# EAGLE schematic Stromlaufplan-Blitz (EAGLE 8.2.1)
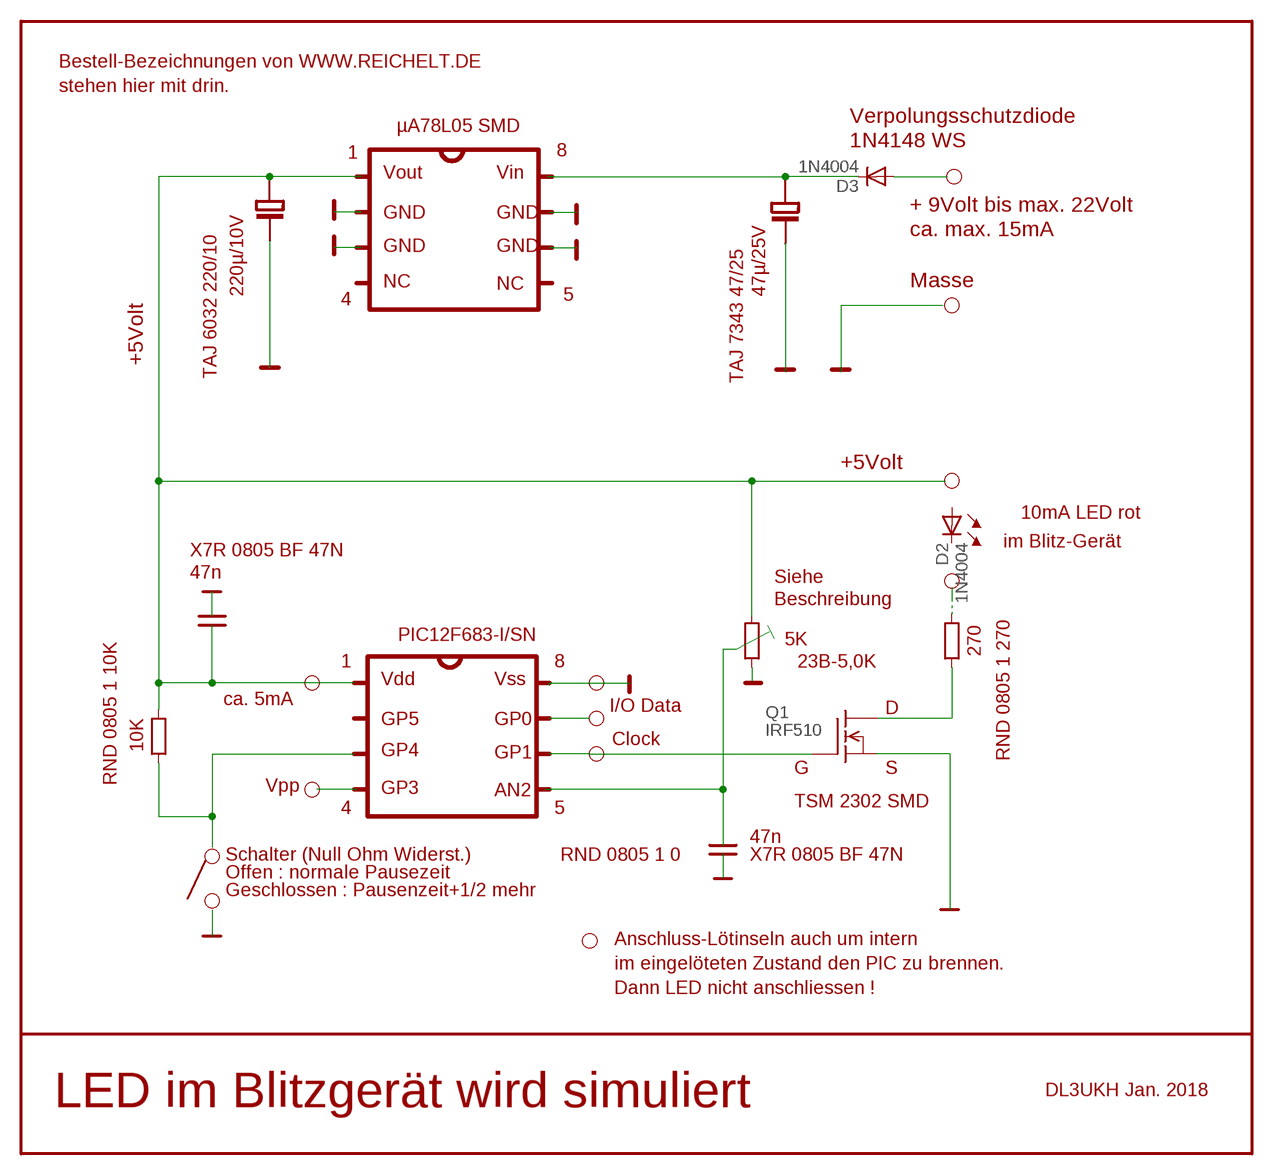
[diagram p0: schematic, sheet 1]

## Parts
D2  1N4004  [DO41-10]
D3  1N4004  [DO41-10]
Q1  IRF510  [TO220]

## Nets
N$5: Q1.1(G)
N$8: Q1.2(D)
N$11: D3.A
N$13: Q1.3(S)
N$35: D3.C
Unconnected: D2.A D2.C

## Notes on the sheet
- Bestell-Bezeichnungen von WWW.REICHELT.DE
- stehen hier mit drin.
- Verpolungsschutzdiode
- µA78L05 SMD
- 1N4148 WS
- 1 | 8
- Vout | Vin
- + 9Volt bis max. 22Volt
- GND | GND
- ca. max. 15mA
- GND | GND
- NC | NC | Masse
- 220µ/10V | 5 | 47µ/25V
- 4
- +5Volt
- TAJ 6032 220/10 | TAJ 7343 47/25
- +5Volt
- 10mA LED rot
- im Blitz-Gerät
- X7R 0805 BF 47N
- 47n | Siehe
- Beschreibung
- PIC12F683-I/SN | 5K
- 23B-5,0K | 270
- 1 | 8
- Vdd | Vss
- ca. 5mA
- I/O Data | D
- GP5 | GP0
- Clock
- 10K | GP4
- GP1 | RND 0805 1 270
- G | S
- RND 0805 1 10K
- Vpp | GP3 | AN2
- TSM 2302 SMD
- 4 | 5
- RND 0805 1 0 | 47n
- Schalter (Null Ohm Widerst.) | X7R 0805 BF 47N
- Offen : normale Pausezeit
- Geschlossen : Pausenzeit+1/2 mehr
- Anschluss-Lötinseln auch um intern
- im eingelöteten Zustand den PIC zu brennen.
- Dann LED nicht anschliessen !
- DL3UKH Jan. 2018
- LED im Blitzgerät wird simuliert

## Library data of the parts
D2 D3 = diode:1N4004: DIODE
Q1 = transistor-fet:IRF510: N-Channel Enhancement MOSFET (HEXFET); 100V; 5,6A; 0,54Ohm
